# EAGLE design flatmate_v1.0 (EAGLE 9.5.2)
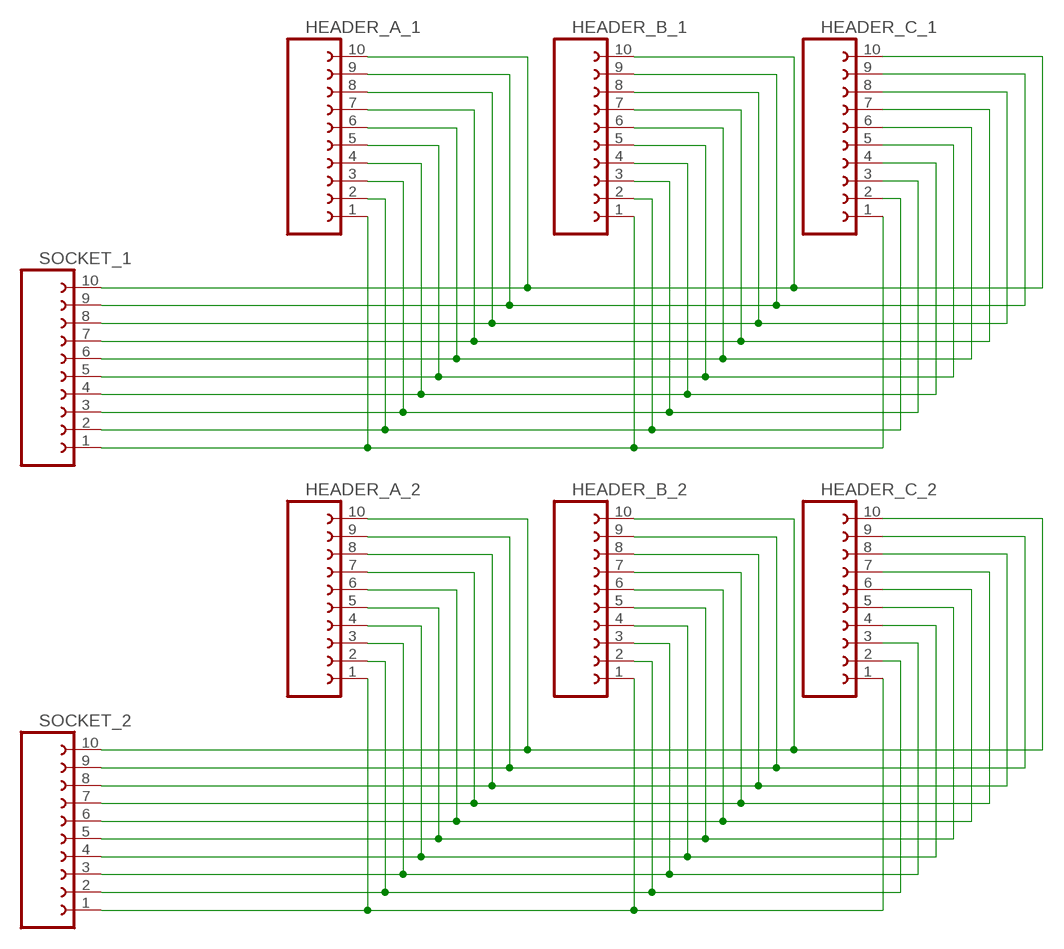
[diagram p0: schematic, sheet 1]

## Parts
HEADER_A_1  2MM_HEADER_1X10_SMD_B_DEV  [2MM_HEADER_1X10_SMD_B]
HEADER_A_2  2MM_HEADER_1X10_SMD_B_DEV  [2MM_HEADER_1X10_SMD_B]
HEADER_B_1  2MM_HEADER_1X10_SMD_B_DEV  [2MM_HEADER_1X10_SMD_B]
HEADER_B_2  2MM_HEADER_1X10_SMD_B_DEV  [2MM_HEADER_1X10_SMD_B]
HEADER_C_1  2MM_HEADER_1X10_SMD_B_DEV  [2MM_HEADER_1X10_SMD_B]
HEADER_C_2  2MM_HEADER_1X10_SMD_B_DEV  [2MM_HEADER_1X10_SMD_B]
SOCKET_1  2MM_SOCKET_1X10_SMD_A_DEV  [2MM_SOCKET_1X10_SMD_A]
SOCKET_2  2MM_SOCKET_1X10_SMD_A_DEV  [2MM_SOCKET_1X10_SMD_A]

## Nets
N$1: HEADER_A_1.1 HEADER_B_1.1 HEADER_C_1.1 SOCKET_1.1
N$2: HEADER_A_1.2 HEADER_B_1.2 HEADER_C_1.2 SOCKET_1.2
N$3: HEADER_A_1.3 HEADER_B_1.3 HEADER_C_1.3 SOCKET_1.3
N$4: HEADER_A_1.5 HEADER_B_1.5 HEADER_C_1.5 SOCKET_1.5
N$5: HEADER_A_1.4 HEADER_B_1.4 HEADER_C_1.4 SOCKET_1.4
N$6: HEADER_A_2.1 HEADER_B_2.1 HEADER_C_2.1 SOCKET_2.1
N$7: HEADER_A_1.6 HEADER_B_1.6 HEADER_C_1.6 SOCKET_1.6
N$8: HEADER_A_2.2 HEADER_B_2.2 HEADER_C_2.2 SOCKET_2.2
N$9: HEADER_A_2.3 HEADER_B_2.3 HEADER_C_2.3 SOCKET_2.3
N$10: HEADER_A_1.7 HEADER_B_1.7 HEADER_C_1.7 SOCKET_1.7
N$11: HEADER_A_2.4 HEADER_B_2.4 HEADER_C_2.4 SOCKET_2.4
N$12: HEADER_A_2.5 HEADER_B_2.5 HEADER_C_2.5 SOCKET_2.5
N$13: HEADER_A_1.8 HEADER_B_1.8 HEADER_C_1.8 SOCKET_1.8
N$14: HEADER_A_2.6 HEADER_B_2.6 HEADER_C_2.6 SOCKET_2.6
N$15: HEADER_A_2.7 HEADER_B_2.7 HEADER_C_2.7 SOCKET_2.7
N$16: HEADER_A_1.9 HEADER_B_1.9 HEADER_C_1.9 SOCKET_1.9
N$17: HEADER_A_2.8 HEADER_B_2.8 HEADER_C_2.8 SOCKET_2.8
N$18: HEADER_A_2.9 HEADER_B_2.9 HEADER_C_2.9 SOCKET_2.9
N$19: HEADER_A_1.10 HEADER_B_1.10 HEADER_C_1.10 SOCKET_1.10
N$20: HEADER_A_2.10 HEADER_B_2.10 HEADER_C_2.10 SOCKET_2.10

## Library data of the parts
HEADER_A_1 HEADER_A_2 HEADER_B_1 HEADER_B_2 HEADER_C_1 HEADER_C_2 = crazyflie:2MM_HEADER_1X10_SMD_B_DEV: 2mm header pin, alternating SMD pads (1x10)
SOCKET_1 SOCKET_2 = crazyflie:2MM_SOCKET_1X10_SMD_A_DEV: 2mm header pin socket, alternating SMD pads (1x10)

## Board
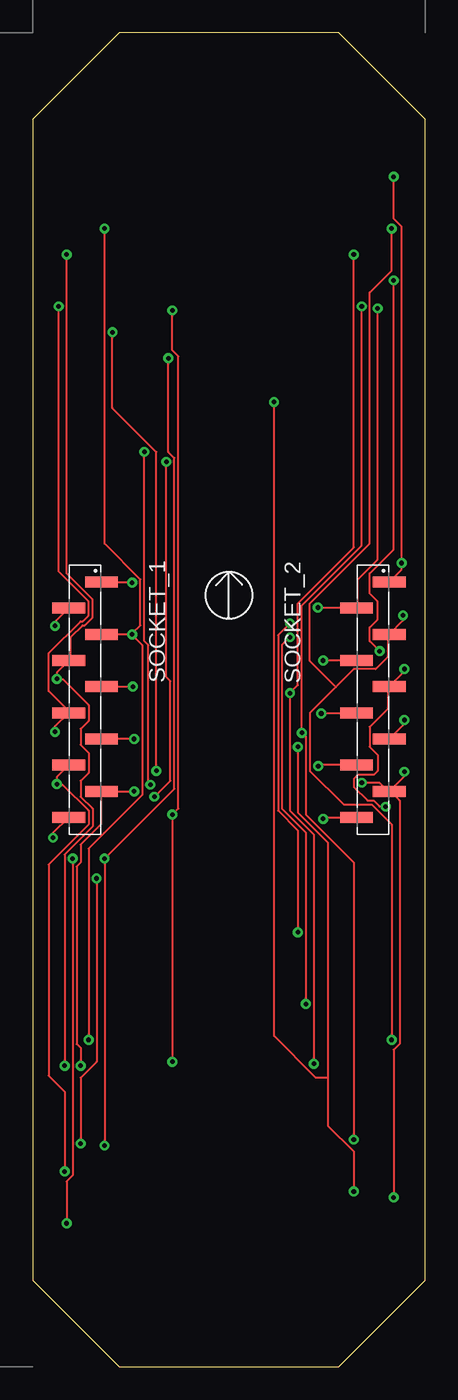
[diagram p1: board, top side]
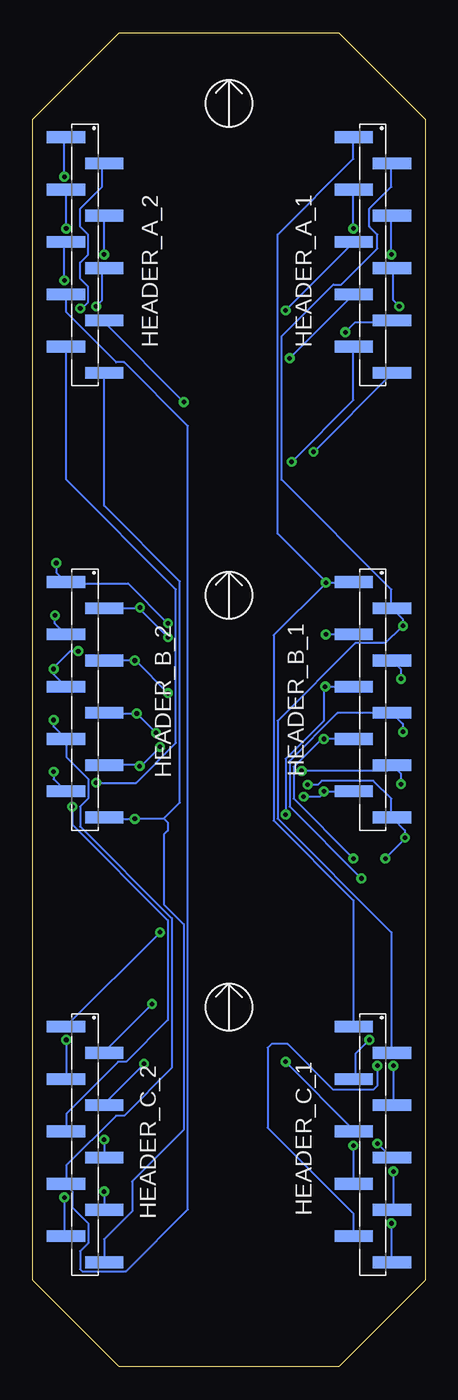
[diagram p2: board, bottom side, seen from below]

Size 30 x 102 mm. Coordinates in mm from the lower left corner, seen from the top.
Outline: 30,6.6 30,95.4 23.4,102 6.6,102 0,95.4 0,6.6 6.6,0 23.4,0 30,6.6
Copper layers (1*16): Top 0.035mm / dielectric 1.5mm / Bottom 0.035mm
Design rules "default": minimum track width 6mil, minimum drill 0.35mm, track to track 6mil, track to pad 6mil, pad to pad 6mil, via to via 6mil, smd to smd 6mil, copper to edge 40mil, drill to drill 6mil, minimum pad ring 10mil, minimum via ring 8mil, stop-mask expansion 4mil, vias tented up to drill 0mil, thermal gap 10mil

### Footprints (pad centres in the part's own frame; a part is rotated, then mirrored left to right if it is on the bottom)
2MM_HEADER_1X10_SMD_B = smd 0.9 x 2.92: 1 -1,-1.46; 2 1,1.46; 3 3,-1.46; 4 5,1.46; 5 7,-1.46; 6 9,1.46; 7 11,-1.46; 8 13,1.46; 9 15,-1.46; 10 17,1.46
2MM_SOCKET_1X10_SMD_A = smd 0.85 x 2.5: 1 -1,1.25; 2 1,-1.25; 3 3,1.25; 4 5,-1.25; 5 7,1.25; 6 9,-1.25; 7 11,1.25; 8 13,-1.25; 9 15,1.25; 10 17,-1.25

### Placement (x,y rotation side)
HEADER_A_1  4,93 270 bottom
HEADER_A_2  26,93 270 bottom
HEADER_B_1  4,59 270 bottom
HEADER_B_2  26,59 270 bottom
HEADER_C_1  4,25 270 bottom
HEADER_C_2  26,25 270 bottom
SOCKET_1  4,59 270 top
SOCKET_2  26,59 270 top

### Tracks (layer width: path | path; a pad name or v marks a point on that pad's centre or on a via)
N$1  (via drill 0.35)
  Top 0.152: SOCKET_1.1 7.6,60 v7.6,59.95
  Bottom 0.152: v7.6,59.95 5.51,59.95 HEADER_B_1.1 | HEADER_C_1.1 5.49,26.06 5.49,35.66 11.58,41.76 11.58,55.93 7.62,59.89 v7.6,59.95 | HEADER_A_1.1 5.49,93.88 5.49,92.35 11.28,86.56 11.28,63.7 7.62,60.05 v7.6,59.95
N$2  (via drill 0.35)
  Top 0.152: v1.7,56.65 1.7,56.95 SOCKET_1.2
  Bottom 0.152: HEADER_C_1.2 2.59,24.08 2.59,33.22 11.28,41.91 11.28,49.38 5.34,55.32 3.05,55.32 1.83,56.54 v1.7,56.65 1.7,57.16 HEADER_B_1.2 2.59,58.06 2.59,59.44 10.98,67.82 10.98,78.79 7.01,82.75 6.4,82.75 3.66,85.5 3.66,86.56 4.27,87.17 4.27,88.54 2.59,90.22 2.59,91.9 HEADER_A_1.2
N$3  (via drill 0.35)
  Top 0.152: v7.6,56 SOCKET_1.3 | v4.27,24.99 4.27,39.62 8.38,43.74 8.38,55.17 7.62,55.93 v7.6,56 | v5.49,87.02 5.49,62.94 8.23,60.2 8.23,56.69 7.62,56.08 v7.6,56
  Bottom 0.152: HEADER_B_1.3 v7.6,56 | v4.27,24.99 5.34,23.93 5.34,22.1 HEADER_C_1.3 | v5.49,87.02 5.49,89.92 HEADER_A_1.3
N$4  (via drill 0.35)
  Top 0.152: SOCKET_1.5 v7.65,52 | v10.67,23.32 v10.67,42.22 11.13,42.67 11.13,77.27 10.67,77.72 v10.67,80.77
  Bottom 0.152: HEADER_B_1.5 v7.65,52 7.77,51.97 7.77,49.38 10.67,46.48 v10.67,42.22 | v10.67,23.32 5.49,18.14 HEADER_C_1.5 | v10.67,80.77 5.49,85.95 HEADER_A_1.5
N$5  (via drill 0.35)
  Top 0.152: v2.44,23.01 2.44,39.17 4.57,41.3 4.57,42.67 3.66,43.59 3.66,44.81 4.27,45.41 4.27,46.94 3.66,47.55 3.66,48.77 4.27,49.38 4.27,50.6 2.29,52.58 1.98,52.58 v1.85,52.6 1.85,53.1 SOCKET_1.4 2.9,54.1 2.9,55.78 3.81,56.69 3.96,56.69 4.57,57.3 4.57,58.67 2.59,60.66 v2.59,85.04
  Bottom 0.152: v1.85,52.6 1.85,53.31 HEADER_B_1.4 | v2.44,23.01 2.44,20.12 HEADER_C_1.4 | v2.59,85.04 2.59,87.94 HEADER_A_1.4
N$6  (via drill 0.35)
  Top 0.152: SOCKET_2.1 28.2,60.95 v28.2,61.45 28.2,61.57 28.2,87.17 27.59,87.78 v27.59,90.98 | v20.27,33.22 20.27,41 18.75,42.52 18.75,55.93 v19.66,56.84
  Bottom 0.152: v28.2,61.45 28.2,60.74 HEADER_B_2.1 27.43,59.89 22.71,59.89 v19.66,56.84 | v20.27,33.22 27.43,26.06 HEADER_C_2.1 | v27.59,90.98 27.59,93.88 HEADER_A_2.1
N$7  (via drill 0.35)
  Top 0.152: v1.7,48.55 1.7,48.95 SOCKET_1.6 2.75,50.14 1.22,51.66 1.22,54.56 3.66,57 3.81,57 4.27,57.45 4.27,58.52 1.98,60.81 v1.98,81.08 | v3.66,17.07 3.66,22.1 4.88,23.32 v4.88,37.34
  Bottom 0.152: v1.7,48.55 1.7,49.16 HEADER_B_1.6 2.59,49.99 6.71,49.99 10.36,46.33 10.36,42.82 v4.88,37.34 | v3.66,17.07 2.59,16 HEADER_C_1.6 | v1.98,81.08 2.44,81.53 2.44,83.97 HEADER_A_1.6
N$8  (via drill 0.35)
  Top 0.152: v21.8,58.05 24.7,58.05 SOCKET_2.2 24.84,58.06 24.84,60.2 26.37,61.72 v26.37,80.92 | v20.88,27.74 20.88,40.84 19.05,42.67 19.05,55.17 v19.66,55.78
  Bottom 0.152: HEADER_B_2.2 21.85,58 v21.8,58.05 21.8,57.91 v19.66,55.78 | v20.88,27.74 24.54,24.08 HEADER_C_2.2 | v26.37,80.92 26.22,80.92 25.76,81.38 25.76,82.6 26.37,83.21 26.37,84.43 25.76,85.04 25.76,86.56 26.37,87.17 26.37,88.54 24.69,90.22 24.69,91.9 HEADER_A_2.2
N$9  (via drill 0.35)
  Top 0.152: v28.3,57.45 28.3,57.05 SOCKET_2.3 27.13,55.93 27.13,54.25 26.22,53.34 24.54,53.34 23.17,51.97 | v27.43,24.99 27.43,41.45 25.91,42.98 23.78,42.98 21.19,45.57 21.19,49.99 23.17,51.97 | v27.43,87.02 27.43,83.82 25.76,82.14 25.76,62.94 21.19,58.37 21.19,53.95 23.17,51.97
  Bottom 0.152: HEADER_B_2.3 28.3,56.84 v28.3,57.45 | v27.43,24.99 27.43,22.1 HEADER_C_2.3 | v27.43,87.02 27.43,89.92 HEADER_A_2.3
N$10  (via drill 0.35)
  Top 0.152: v7.75,48 SOCKET_1.7 | v5.49,16.92 v5.49,38.86 10.82,44.2 10.82,69.49 10.36,69.95 v10.36,77.11
  Bottom 0.152: HEADER_B_1.7 v7.75,48 7.77,47.85 8.08,47.85 10.06,45.87 10.06,43.43 v5.49,38.86 | v5.49,16.92 5.49,14.02 HEADER_C_1.7 | v10.36,77.11 5.49,81.99 HEADER_A_1.7
N$11  (via drill 0.35)
  Top 0.152: SOCKET_2.4 v22.2,54 | v21.49,23.16 21.49,40.69 19.66,42.52 v19.66,51.51 20.27,52.12 20.27,58.37 24.54,62.64 v24.54,85.04
  Bottom 0.152: HEADER_B_2.4 v22.2,54 22.1,53.95 v19.66,51.51 | v21.49,23.16 24.54,20.12 HEADER_C_2.4 | v24.54,85.04 24.54,87.94 HEADER_A_2.4
N$12  (via drill 0.35)
  Top 0.152: v28.4,53.35 28.45,53.35 28.45,53.2 SOCKET_2.5 27.13,51.97 27.13,50.29 25.76,48.92 25.76,47.4 26.37,46.79 26.37,45.57 26.06,45.26 24.84,45.26 24.54,44.96 24.54,44.35 25.6,43.28 26.06,43.28 26.52,42.82 v26.98,42.82 | v27.59,83.06 27.59,62.48 25.76,60.66 25.76,59.13 26.37,58.52 26.37,57.15 25.76,56.54 25.76,55.47 v26.52,54.71
  Bottom 0.152: HEADER_B_2.5 28.4,52.94 v28.4,53.35 28.35,53.49 27.13,54.71 v26.52,54.71 | v26.98,42.82 26.98,41.45 19.66,34.14 19.66,26.52 22.86,23.32 23.47,23.32 27.43,19.36 27.43,18.14 HEADER_C_2.5 | v27.59,83.06 27.59,85.95 HEADER_A_2.5
N$13  (via drill 0.35)
  Top 0.152: SOCKET_1.8 1.85,45.1 v1.85,44.55 1.98,44.5 2.29,44.5 4.27,42.52 4.27,41.45 1.22,38.41 1.22,22.25 2.44,21.03 v2.44,14.94 | v6.1,79.1 6.1,73.3 9.45,69.95 v9.45,45.57
  Bottom 0.152: v1.85,44.55 1.85,45.31 HEADER_B_1.8 2.59,45.87 2.9,45.57 v9.45,45.57 | v2.44,14.94 2.44,12.04 HEADER_C_1.8 | v6.1,79.1 5.34,79.86 2.59,79.86 HEADER_A_1.8
N$14  (via drill 0.35)
  Top 0.152: v22.05,49.95 22.1,50 SOCKET_2.6 | v24.54,17.37 24.54,38.56 20.88,42.22 20.88,48.16 v20.58,48.46 20.58,58.22 25.15,62.79 v25.15,81.08
  Bottom 0.152: HEADER_B_2.6 24.49,49.95 v22.05,49.95 21.95,49.84 v20.58,48.46 | v24.54,17.37 HEADER_C_2.6 | v25.15,81.08 24.69,81.53 24.69,83.97 HEADER_A_2.6
N$15  (via drill 0.35)
  Top 0.152: v28.4,49.45 28.4,49.15 SOCKET_2.7
  Bottom 0.152: v28.4,49.45 28.4,48.94 HEADER_B_2.7 27.43,47.85 27.43,46.63 25.76,44.96 25.76,43.43 26.37,42.82 26.37,41.3 19.36,34.29 19.36,22.86 23.01,19.2 23.62,19.2 27.43,15.39 27.43,14.02 HEADER_C_2.7 27.43,13.87 26.98,13.41 26.98,12.19 25.76,10.97 25.76,9.45 26.37,8.84 26.37,7.47 26.22,7.32 22.86,7.32 18.14,12.04 18.14,71.93 23.01,76.81 23.62,76.81 27.43,80.62 27.43,81.99 HEADER_A_2.7
N$16  (via drill 0.35)
  Top 0.152: v7.75,44 SOCKET_1.9 5.18,43.89 5.18,41.45 3.66,39.93 3.66,38.56 3.36,38.25 3.36,24.69 3.66,24.38 v3.66,23.01 | v10.21,69.19 10.21,52.73 10.52,52.43 10.52,44.81 v9.3,43.59
  Bottom 0.152: HEADER_B_1.9 v7.75,44 7.77,43.89 8.08,43.59 v9.3,43.59 | v3.66,23.01 3.66,21.49 3.96,21.18 7.01,21.18 10.52,24.69 11.74,24.69 12.04,24.38 12.04,18.29 5.49,11.73 5.49,10.06 HEADER_C_1.9 | v10.21,69.19 5.49,73.91 5.49,77.88 HEADER_A_1.9
N$17  (via drill 0.35)
  Top 0.152: SOCKET_2.8 21.85,46 21.8,45.95 v21.83,45.92 | v24.54,13.41 24.54,16.46 22.56,18.44 22.56,22.1 | 22.56,22.1 22.56,40.08 20.27,42.37 v20.27,47.4 | v18.44,73.76 18.44,25.3 21.64,22.1 22.56,22.1
  Bottom 0.152: HEADER_B_2.8 21.9,46 v21.83,45.92 21.8,45.87 v20.27,47.4 | v24.54,13.41 24.54,12.04 HEADER_C_2.8 | v18.44,73.76 24.54,79.86 HEADER_A_2.8
N$18  (via drill 0.35)
  Top 0.152: SOCKET_2.9 28.4,45.15 v28.4,45.5 | v27.59,12.95 27.59,24.23 28.04,24.69 28.04,43.28 27.28,44.04 SOCKET_2.9 | v25.15,44.65 26.52,44.65 27.13,44.04 SOCKET_2.9
  Bottom 0.152: v28.4,45.5 28.4,44.94 HEADER_B_2.9 | v27.59,12.95 27.59,10.06 HEADER_C_2.9 | v25.15,44.65 22.1,44.65 19.05,47.7 19.05,59.44 27.43,67.82 27.43,77.88 HEADER_A_2.9
N$19  (via drill 0.35)
  Top 0.152: v1.55,40.45 1.55,40.8 SOCKET_1.10 | v2.59,10.97 2.59,14.17 3.05,14.63 v3.05,38.86 | v8.54,69.95 8.54,55.47 8.84,55.17 8.84,44.65 v8.99,44.5
  Bottom 0.152: v2.59,10.97 2.59,8.08 HEADER_C_1.10 | v3.05,38.86 1.53,40.39 v1.55,40.45 1.55,41.01 HEADER_B_1.10 2.59,42.06 2.59,43.43 3.96,44.81 7.93,44.81 8.23,44.5 v8.99,44.5 | v8.54,69.95 2.59,75.89 HEADER_A_1.10
N$20  (via drill 0.35)
  Top 0.152: v22.2,41.9 22.3,42 SOCKET_2.10
  Bottom 0.152: HEADER_B_2.10 24.44,41.9 v22.2,41.9 22.1,41.91 19.97,41.91 | 19.97,41.91 19.66,41.6 19.66,41 19.97,40.69 19.97,35.36 18.44,33.83 18.44,18.14 22.41,14.17 22.41,11.89 24.54,9.75 24.54,8.08 HEADER_C_2.10 | 19.97,41.91 18.75,43.13 18.75,60.05 24.54,65.84 24.54,75.89 HEADER_A_2.10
